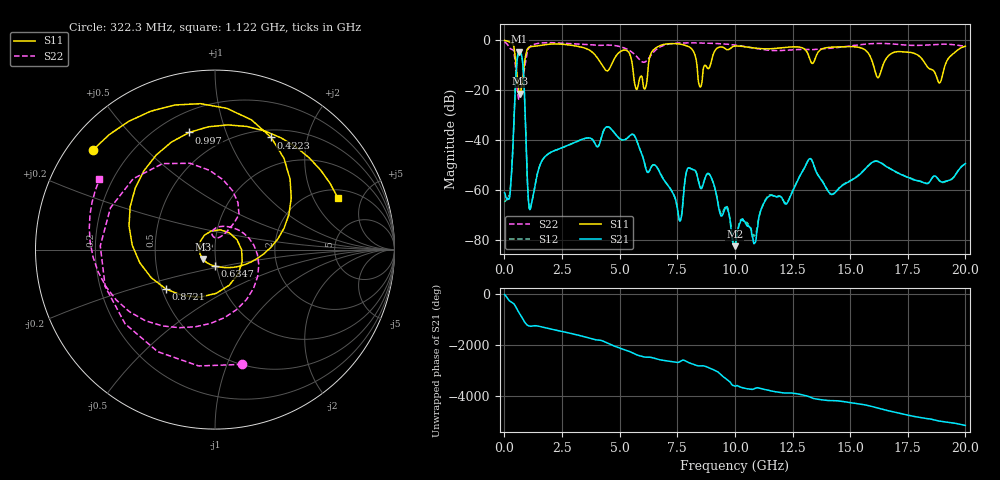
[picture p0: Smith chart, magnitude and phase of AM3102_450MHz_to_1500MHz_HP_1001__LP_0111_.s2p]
!Agilent Technologies,E8364B,MY43040894,A.07.50.67
!Agilent E8364B: A.07.50.67
!Date: Thursday, January 11, 2018 06:02:59
!Correction: S11(Full 2 Port(1,2))
!S21(Full 2 Port(1,2))
!S12(Full 2 Port(1,2))
!S22(Full 2 Port(1,2))
!S2P File: Measurements: S11, S21, S12, S22:
# Hz S  dB  R 50
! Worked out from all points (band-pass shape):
!   1601 points, 10 MHz to 20 GHz, reference 50 ohm
!   highest |S21| = -4.54 dB at 647.2 MHz (marker M1); lowest = -82.4 dB at 9.993 GHz (marker M2)
!   |S21| within 3 dB of the highest: 557.2 MHz to 777.1 MHz (219.9 MHz wide, 33 % of centre)
!   lowest |S11| = -21.3 dB at 672.2 MHz (marker M3), VSWR 1.19, Z = 43.4 - j4.61 ohm
!   |S11| at or under -10 dB: 5.554 GHz to 6.246 GHz (692.2 MHz wide, 11.7 % of centre); 16.01 GHz to 16.42 GHz (410.9 MHz wide, 2.53 % of centre); 18.3 GHz to 19.12 GHz (816.8 MHz wide, 4.37 % of centre)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
!   |S22| runs from -23.8 to -0.6 dB; largest |S21 - S12| = 0.0016
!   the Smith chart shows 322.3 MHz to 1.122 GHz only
!   S11 on the Smith chart (normalised r, x): 322.3 MHz: 0.07, +0.35; 422.3 MHz: 0.59, +1.45; 634.7 MHz: 0.98, -0.18; 872.1 MHz: 0.53, -0.26; 997 MHz: 0.32, +0.75; 1.122 GHz: 2.45, +3.15
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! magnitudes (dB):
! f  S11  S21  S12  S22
! 10 MHz  -0.1  -61.1  -64.3  -0.6
! 322.3 MHz  -1.1  -51.3  -51.1  -3.6
! 422.3 MHz  -3.1  -29.9  -29.9  -5.0
! 634.7 MHz  -20.7  -4.6  -4.6  -23.8
! 647.2 MHz  -21.1  -4.5  -4.5  -23.6
! 672.2 MHz  -21.3  -4.6  -4.6  -22.9
! 872.1 MHz  -9.1  -21.9  -21.9  -11.0
! 997 MHz  -3.5  -55.8  -55.9  -4.6
! 1.122 GHz  -2.6  -67.6  -67.7  -2.5
! 3.346 GHz  -2.7  -39.7  -39.7  -1.6
! 5.732 GHz  -19.6  -39.8  -39.8  -6.4
! 6.682 GHz  -2.4  -51.8  -51.6  -3.1
! 7.619 GHz  -1.5  -72.4  -72.0  -1.1
! 7.969 GHz  -2.4  -51.1  -51.1  -1.0
! 8.893 GHz  -10.9  -53.5  -53.7  -1.2
! 9.993 GHz  -2.3  -82.4  -81.3  -1.9
! 10.01 GHz  -2.3  -82.2  -81.4  -1.9
! 13.34 GHz  -9.2  -48.0  -48.0  -3.7
! 14.19 GHz  -2.7  -61.6  -61.7  -3.1
! 16.68 GHz  -6.1  -51.0  -51.1  -1.3
! 18.88 GHz  -17.1  -56.1  -56.3  -1.6
! 20 GHz  -2.4  -49.3  -49.5  -2.3
